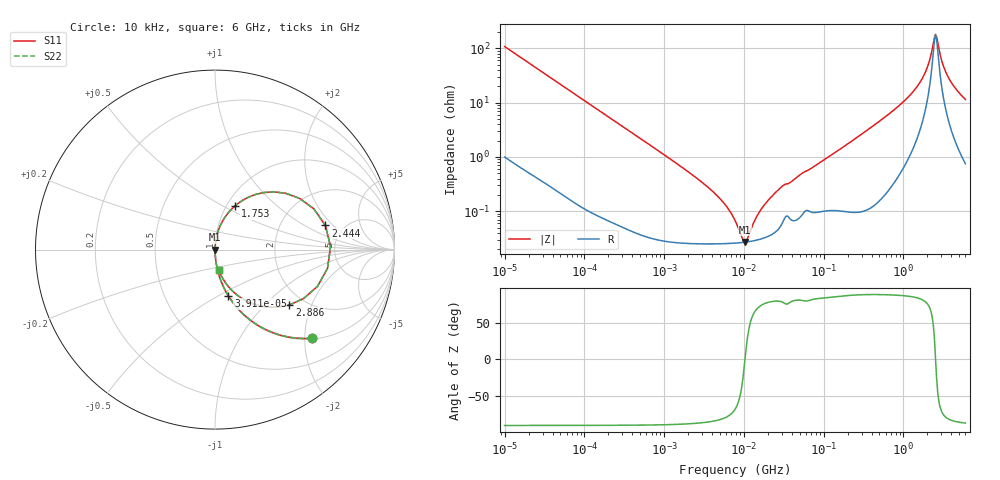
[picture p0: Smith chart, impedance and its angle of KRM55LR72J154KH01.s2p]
!Murata Part Number: KRM55LR72J154KH01
!These Parameters are Measured in Series Mode Connection
!Data Generated on Jan 08, 2026
!  o--ll--o
!Port1  Port2
!  o------o
!Operation Temp=25[degC], DC Bias Voltage=0[V]
!Freq. Start=10[kHz] Stop=6[GHz] 401[Steps]
# Hz S RI R 50
!Freq.(Hz) S11(Real) S11(Imag) S21(Real) S21(Imag) S12(Real) S12(Imag) S22(Real) S22(Imag)
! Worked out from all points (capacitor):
!   401 points, 10 kHz to 6 GHz, reference 50 ohm
!   read as one part in series: C = 147 nF near 10.69 kHz
!   lowest |Z| = 27.1 mohm at 10.45 MHz (marker M1)
!   series resonance near 10.34 MHz, so ESL is about 1.6 nH
!   S11 on the Smith chart (normalised r, x): 10 kHz: 1.02, -2.17; 39.11 kHz: 1.01, -0.56; 1.753 GHz: 1.09, +0.57; 2.444 GHz: 3.63, +1.62; 2.886 GHz: 1.67, -1.41; 6 GHz: 1.02, -0.23
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10000  0.5395 -0.4939  0.4605 0.4939  0.4605 0.4939  0.5395 -0.4939
20787  0.2171 -0.4076  0.7829 0.4076  0.7829 0.4076  0.2171 -0.4076
39108  0.0745 -0.2577  0.9255 0.2577  0.9255 0.2577  0.0745 -0.2577
92862  0.0149 -0.1162  0.9851 0.1162  0.9851 0.1162  0.0149 -0.1162
862344  0.000455 -0.0128  0.9995 0.0128  0.9995 0.0128  0.000455 -0.0128
3982613  0.000255 -0.00237  0.9997 0.00237  0.9997 0.00237  0.000255 -0.00237
5936256  0.000255 -0.00125  0.9997 0.00125  0.9997 0.00125  0.000255 -0.00125
7745967  0.000259 -0.000628  0.9997 0.000628  0.9997 0.000628  0.000259 -0.000628
9456880  0.000265 -0.000191  0.9997 0.000191  0.9997 0.000191  0.000265 -0.000191
1.044922e7  0.00027 2.35e-05  0.9997 -2.35e-05  0.9997 -2.35e-05  0.00027 2.35e-05
1.506549e7  0.000298 0.000829  0.9997 -0.000829  0.9997 -0.000829  0.000298 0.000829
2.172113e7  0.000366 0.00175  0.9996 -0.00175  0.9996 -0.00175  0.000366 0.00175
7.193098e7  0.000991 0.00626  0.999 -0.00626  0.999 -0.00626  0.000991 0.00626
6.67969e8  0.00641 0.0622  0.9936 -0.0622  0.9936 -0.0622  0.00641 0.0622
1.215551e9  0.0287 0.1323  0.9713 -0.1323  0.9713 -0.1323  0.0287 0.1323
1.752557e9  0.1114 0.2433  0.8886 -0.2433  0.8886 -0.2433  0.1114 0.2433
2.139659e9  0.3248 0.322  0.6752 -0.322  0.6752 -0.322  0.3248 0.322
2.44414e9  0.6149 0.1344  0.3851 -0.1344  0.3851 -0.1344  0.6149 0.1344
2.612262e9  0.6271 -0.1039  0.3729 0.1039  0.3729 0.1039  0.6271 -0.1039
2.886376e9  0.4148 -0.3085  0.5852 0.3085  0.5852 0.3085  0.4148 -0.3085
3.643096e9  0.1163 -0.2476  0.8837 0.2476  0.8837 0.2476  0.1163 -0.2476
6e9  0.0201 -0.1114  0.9799 0.1114  0.9799 0.1114  0.0201 -0.1114
